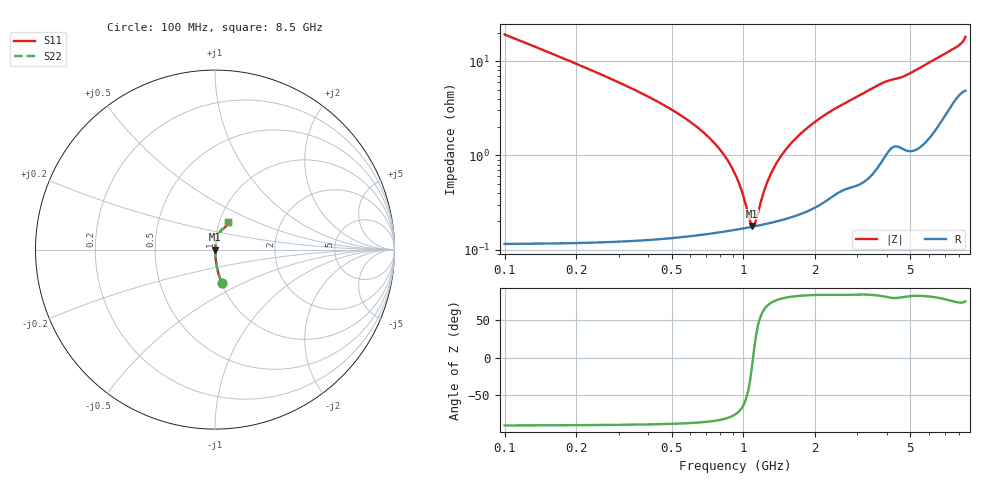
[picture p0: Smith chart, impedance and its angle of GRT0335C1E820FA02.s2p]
!Murata Part Number: GRT0335C1E820FA02
!These Parameters are Measured in Series Mode Connection
!Data Generated on Jun 19, 2026
!  o--ll--o
!Port1  Port2
!  o------o
!Operation Temp=25[degC], DC Bias Voltage=0[V]
!Freq. Start=100[MHz] Stop=9[GHz] 401[Steps]
# Hz S RI R 50
!Freq.(Hz) S11(Real) S11(Imag) S21(Real) S21(Imag) S12(Real) S12(Imag) S22(Real) S22(Imag)
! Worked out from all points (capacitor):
!   401 points, 100 MHz to 8.5 GHz, reference 50 ohm
!   read as one part in series: C = 82 pF near 142 MHz
!   lowest |Z| = 178 mohm at 1.087 GHz (marker M1)
!   series resonance near 1.097 GHz, so ESL is about 260 pH
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1e8  0.0367 -0.1852  0.9633 0.1852  0.9633 0.1852  0.0367 -0.1852
2.05e8  0.00942 -0.0904  0.9906 0.0904  0.9906 0.0904  0.00942 -0.0904
3.1e8  0.00451 -0.0572  0.9955 0.0572  0.9955 0.0572  0.00451 -0.0572
7.09e8  0.00171 -0.0158  0.9983 0.0158  0.9983 0.0158  0.00171 -0.0158
8.35e8  0.00165 -0.00972  0.9984 0.00972  0.9984 0.00972  0.00165 -0.00972
9.4e8  0.00166 -0.00546  0.9983 0.00546  0.9983 0.00546  0.00166 -0.00546
1.045e9  0.00171 -0.00172  0.9983 0.00172  0.9983 0.00172  0.00171 -0.00172
1.087e9  0.00174 -0.000335  0.9983 0.000335  0.9983 0.000335  0.00174 -0.000335
1.129e9  0.00178 0.000996  0.9982 -0.000996  0.9982 -0.000996  0.00178 0.000996
1.234e9  0.00188 0.00413  0.9981 -0.00413  0.9981 -0.00413  0.00188 0.00413
1.297e9  0.00195 0.0059  0.998 -0.0059  0.998 -0.0059  0.00195 0.0059
1.381e9  0.00206 0.00815  0.9979 -0.00815  0.9979 -0.00815  0.00206 0.00815
1.507e9  0.00224 0.0114  0.9978 -0.0114  0.9978 -0.0114  0.00224 0.0114
1.738e9  0.00266 0.0168  0.9973 -0.0168  0.9973 -0.0168  0.00266 0.0168
2.053e9  0.00346 0.0237  0.9965 -0.0237  0.9965 -0.0237  0.00346 0.0237
2.914e9  0.00625 0.0399  0.9938 -0.0399  0.9938 -0.0399  0.00625 0.0399
3.733e9  0.0111 0.0554  0.9889 -0.0554  0.9889 -0.0554  0.0111 0.0554
4.3e9  0.0162 0.0617  0.9838 -0.0617  0.9838 -0.0617  0.0162 0.0617
5.707e9  0.0207 0.0861  0.9793 -0.0861  0.9793 -0.0861  0.0207 0.0861
7.114e9  0.0408 0.1123  0.9592 -0.1123  0.9592 -0.1123  0.0408 0.1123
8.08e9  0.0607 0.13  0.9393 -0.13  0.9393 -0.13  0.0607 0.13
8.5e9  0.0721 0.1544  0.9279 -0.1544  0.9279 -0.1544  0.0721 0.1544
